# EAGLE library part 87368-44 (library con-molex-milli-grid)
RECEPTACAL
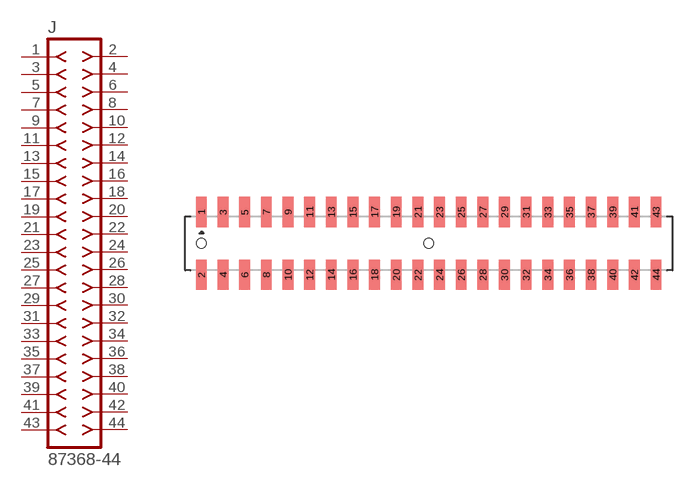
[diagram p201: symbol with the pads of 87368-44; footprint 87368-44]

Designator prefix J

## 87368-44  [87368-44]
1  1  pas
2  2  pas
3  3  pas
4  4  pas
5  5  pas
6  6  pas
7  7  pas
8  8  pas
9  9  pas
10  10  pas
11  11  pas
12  12  pas
13  13  pas
14  14  pas
15  15  pas
16  16  pas
17  17  pas
18  18  pas
19  19  pas
20  20  pas
21  21  pas
22  22  pas
23  23  pas
24  24  pas
25  25  pas
26  26  pas
27  27  pas
28  28  pas
29  29  pas
30  30  pas
31  31  pas
32  32  pas
33  33  pas
34  34  pas
35  35  pas
36  36  pas
37  37  pas
38  38  pas
39  39  pas
40  40  pas
41  41  pas
42  42  pas
43  43  pas
44  44  pas

## Footprint 87368-44 (pad centres in mm)
RECEPTACAL SMD Dual Row, Side Entry
smd 1 x 2.8: 1 -21,2.9; 2 -21,-2.9; 3 -19,2.9; 4 -19,-2.9; 5 -17,2.9; 6 -17,-2.9; 7 -15,2.9; 8 -15,-2.9; 9 -13,2.9; 10 -13,-2.9; 11 -11,2.9; 12 -11,-2.9; 13 -9,2.9; 14 -9,-2.9; 15 -7,2.9; 16 -7,-2.9; 17 -5,2.9; 18 -5,-2.9; 19 -3,2.9; 20 -3,-2.9; 21 -1,2.9; 22 -1,-2.9; 23 1,2.9; 24 1,-2.9; 25 3,2.9; 26 3,-2.9; 27 5,2.9; 28 5,-2.9; 29 7,2.9; 30 7,-2.9; 31 9,2.9; 32 9,-2.9; 33 11,2.9; 34 11,-2.9; 35 13,2.9; 36 13,-2.9; 37 15,2.9; 38 15,-2.9; 39 17,2.9; 40 17,-2.9; 41 19,2.9; 42 19,-2.9; 43 21,2.9; 44 21,-2.9
hole 0.914 at -21,0
hole 0.914 at 0,0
